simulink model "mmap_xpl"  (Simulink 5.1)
settings: Solver=ode45  StartTime=0.0  StopTime=100.0  RelTol=1e-3
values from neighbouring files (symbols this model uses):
  tmp1 = [r0r2clkf r1r3clkf laf ldf ra0f ra1f ra2f ra3f rc0f rc1f rc2f  	      rc3f rd0f rd1f rd2f rd3f]    [createucf_fromvhdl.m]
undefined symbols (not defined in the file or in its folder): Bit, Location, Lower, Width
libraries: xbsIndex_r3 x28, ADlibrary x3, xrbsControl_r3 x1

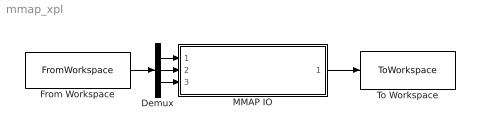
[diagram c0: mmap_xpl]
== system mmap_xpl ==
  Demux : Demux  Outputs=3
  From Workspace : FromWorkspace  InitFcn=init_mmap_program  VariableName=mmap_program  SampleTime=0
  MMAP IO : Subsystem
  To Workspace : ToWorkspace  VariableName=mmap_output  SampleTime=-1  SaveFormat=Structure
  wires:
  From Workspace/1 -> Demux/1
  Demux/1 -> MMAP IO/1(Data Input)
  Demux/2 -> MMAP IO/2(Addr)
  Demux/3 -> MMAP IO/3(Write)
  MMAP IO/1(Data Output) -> To Workspace/1

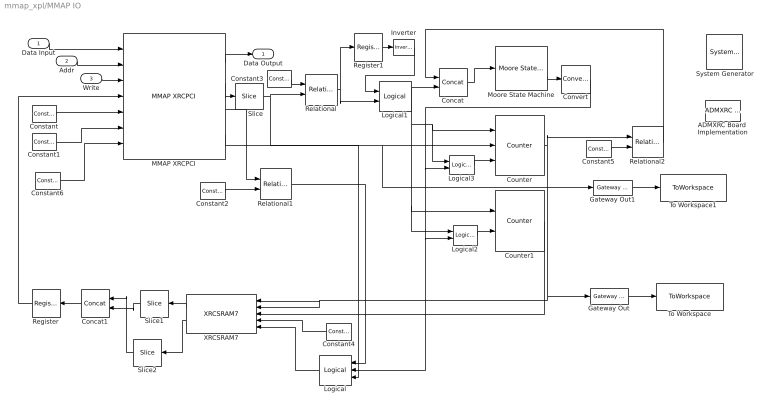
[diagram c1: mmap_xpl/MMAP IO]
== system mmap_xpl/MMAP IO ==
  Data Input : Inport
  Addr : Inport  Port=2
  Write : Inport  Port=3
  " System Generator" : xbsIndex_r3/ System Generator  Tag=genX  xilinxfamily=Virtex2P  part=xc2vp7  speed=-6  package=ff896  synthesis_tool=XST  directory=e:/tmp1  testbench=off  simulink_period=1  sysclk_period=10  incr_netlist=off  trim_vbits=According to Block Masks  dbl_ovrd=According to Block Masks  core_generation=According to Block Masks  run_coregen=off  deprecated_control=off  eval_field=0
  ADMXRC Board  Implementation : ADlibrary/Miscellaneous/ADMXRC Board  Implementation  board=XPL  run_synth=on  make_clean=off  lvds_io_std=3.3v  clock_source=MCLK
  Concat : xbsIndex_r3/Concat  num_inputs=2  explicit_period=off  period=1  dbl_ovrd=off
  Concat1 : xbsIndex_r3/Concat  Orientation=left  num_inputs=2  explicit_period=off  period=1  dbl_ovrd=off
  Constant : xbsIndex_r3/Constant  const=0  arith_type=Unsigned  n_bits=9  bin_pt=0  explicit_period=on  period=1  dbl_ovrd=off
  Constant1 : xbsIndex_r3/Constant  const=0  arith_type=Unsigned  n_bits=1  bin_pt=0  explicit_period=on  period=1  dbl_ovrd=off
  Constant2 : xbsIndex_r3/Constant  const=0  arith_type=Unsigned  n_bits=6  bin_pt=0  explicit_period=on  period=1  dbl_ovrd=off
  Constant3 : xbsIndex_r3/Constant  const=0  arith_type=Unsigned  n_bits=16  bin_pt=0  explicit_period=on  period=1  dbl_ovrd=off
  Constant4 : xbsIndex_r3/Constant  Orientation=left  const=0  arith_type=Unsigned  n_bits=1  bin_pt=0  explicit_period=on  period=1  dbl_ovrd=off
  Constant5 : xbsIndex_r3/Constant  const=0  arith_type=Unsigned  n_bits=16  bin_pt=0  explicit_period=on  period=1  dbl_ovrd=off
  Constant6 : xbsIndex_r3/Constant  const=0  arith_type=Boolean  n_bits=1  bin_pt=0  explicit_period=on  period=1  dbl_ovrd=off
  Convert : xbsIndex_r3/Convert  arith_type=Boolean  n_bits=8  bin_pt=6  quantization=Truncate  overflow=Wrap  latency=0  explicit_period=off  period=1  dbl_ovrd=off  inserted_by_tool=off
  Counter : xbsIndex_r3/Counter  cnt_type=Free Running  n_bits=16  bin_pt=0  arith_type=Unsigned  start_count=0  cnt_to=Inf  cnt_by_val=1  operation=Down  explicit_period=on  period=1  load_pin=on  rst=off  en=on  dbl_ovrd=off  use_rpm=off  gen_core=on
  Counter1 : xbsIndex_r3/Counter  cnt_type=Free Running  n_bits=16  bin_pt=0  arith_type=Unsigned  start_count=0  cnt_to=Inf  cnt_by_val=1  operation=Up  explicit_period=on  period=1  load_pin=off  rst=on  en=on  dbl_ovrd=off  use_rpm=off  gen_core=on
  Gateway Out : xbsIndex_r3/Gateway Out  hdl_port=off  timing_constraint=None  locs_specified=off  LOCs={}  needs_fixed_name=off
  Gateway Out1 : xbsIndex_r3/Gateway Out  hdl_port=off  timing_constraint=None  locs_specified=off  LOCs={}  needs_fixed_name=off
  Inverter : xbsIndex_r3/Inverter  latency=0  explicit_period=on  period=1  en=off  dbl_ovrd=off
  Logical : xbsIndex_r3/Logical  Orientation=left  logical_function=AND  inputs=3  precision=Full  arith_type=Unsigned  n_bits=8  bin_pt=2  align_bp=on  latency=0  explicit_period=off  period=1  en=off  dbl_ovrd=off
  Logical1 : xbsIndex_r3/Logical  logical_function=AND  inputs=2  precision=Full  arith_type=Unsigned  n_bits=8  bin_pt=2  align_bp=on  latency=0  explicit_period=on  period=1  en=off  dbl_ovrd=off
  Logical2 : xbsIndex_r3/Logical  logical_function=OR  inputs=2  precision=Full  arith_type=Unsigned  n_bits=8  bin_pt=2  align_bp=on  latency=0  explicit_period=on  period=1  en=off  dbl_ovrd=off
  Logical3 : xbsIndex_r3/Logical  logical_function=OR  inputs=2  precision=Full  arith_type=Unsigned  n_bits=8  bin_pt=2  align_bp=on  latency=0  explicit_period=on  period=1  en=off  dbl_ovrd=off
  MMAP XRCPCI : ADlibrary/PCI/MMAP XRCPCI  AncestorBlock=ADlibrary/PCI/DWSR XRCPCI  qv132678sdfs=0
  Moore State Machine : xrbsControl_r3/Moore State Machine  next_state_matrix=[0 1 0 1; 1 1 2 2; 0 0 0 0]  output_matrix=[0; 1; 0 ]  n_bits=1  period=1
  Register : xbsIndex_r3/Register  Orientation=left  init=0  reg_only_valid=off  explicit_period=off  period=1  rst=off  en=off  out_en=off  dbl_ovrd=off
  Register1 : xbsIndex_r3/Register  init=0  reg_only_valid=off  explicit_period=on  period=1  rst=off  en=off  out_en=off  dbl_ovrd=off
  Relational : xbsIndex_r3/Relational  mode=a!=b  latency=0  explicit_period=on  period=1  en=off  dbl_ovrd=off
  Relational1 : xbsIndex_r3/Relational  mode=a=b  latency=0  explicit_period=off  period=1  en=off  dbl_ovrd=off
  Relational2 : xbsIndex_r3/Relational  mode=a=b  latency=0  explicit_period=off  period=1  en=off  dbl_ovrd=off
  Slice : xbsIndex_r3/Slice  mode=Lower Bit Location + Width  nbits=16  bit1=0  base1=MSB of Input  bit0=0  base0=LSB of Input  boolean_output=off  explicit_period=off  period=1  dbl_ovrd=off
  Slice1 : xbsIndex_r3/Slice  Orientation=left  mode=Lower Bit Location + Width  nbits=16  bit1=0  base1=MSB of Input  bit0=0  base0=LSB of Input  boolean_output=off  explicit_period=off  period=1  dbl_ovrd=off
  Slice2 : xbsIndex_r3/Slice  Orientation=left  mode=Lower Bit Location + Width  nbits=16  bit1=0  base1=MSB of Input  bit0=16  base0=LSB of Input  boolean_output=off  explicit_period=off  period=1  dbl_ovrd=off
  To Workspace : ToWorkspace  VariableName=simout  SampleTime=-1  SaveFormat=Structure
  To Workspace1 : ToWorkspace  VariableName=simout1  SampleTime=-1  SaveFormat=Structure
  XRCSRAM7 : ADlibrary/Memory/XRCSRAM7  Orientation=left
  Data Output : Outport
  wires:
  MMAP XRCPCI/1 -> Data Output/1
  Write/1 -> MMAP XRCPCI/3
  Addr/1 -> MMAP XRCPCI/2
  Data Input/1 -> MMAP XRCPCI/1
  Constant/1 -> MMAP XRCPCI/5
  Constant1/1 -> MMAP XRCPCI/6
  Constant3/1 -> Relational/1
  MMAP XRCPCI/2 -> Slice/1
  Relational/1 -> Register1/1, Logical1/2
  Slice/1 -> Relational/2, Counter/2, Gateway Out1/1
  Register/1 -> MMAP XRCPCI/4
  MMAP XRCPCI/3 -> Relational1/1
  Constant2/1 -> Relational1/2
  Moore State Machine/2 -> Convert/1
  Counter/1 -> Relational2/1, Gateway Out/1, XRCSRAM7/1, XRCSRAM7/2
  Constant5/1 -> Relational2/2
  Relational2/1 -> Concat/1
  Concat/1 -> Moore State Machine/1
  Logical/1 -> XRCSRAM7/5
  Relational1/1 -> Logical/1
  Convert/1 -> Logical/2, Logical2/2, Logical3/2
  Gateway Out/1 -> To Workspace/1
  Gateway Out1/1 -> To Workspace1/1
  Logical1/1 -> Concat/2, Counter/1, Logical3/1, Counter1/1, Logical2/1
  Register1/1 -> Inverter/1
  Inverter/1 -> Logical1/1
  Logical3/1 -> Counter/3
  Logical2/1 -> Counter1/2
  Constant4/1 -> XRCSRAM7/4
  Counter1/1 -> XRCSRAM7/3
  Concat1/1 -> Register/1
  XRCSRAM7/1 -> Slice1/1
  Slice1/1 -> Concat1/2
  XRCSRAM7/2 -> Slice2/1
  Slice2/1 -> Concat1/1
  Constant6/1 -> MMAP XRCPCI/7
  MMAP XRCPCI/4 -> Logical/3
